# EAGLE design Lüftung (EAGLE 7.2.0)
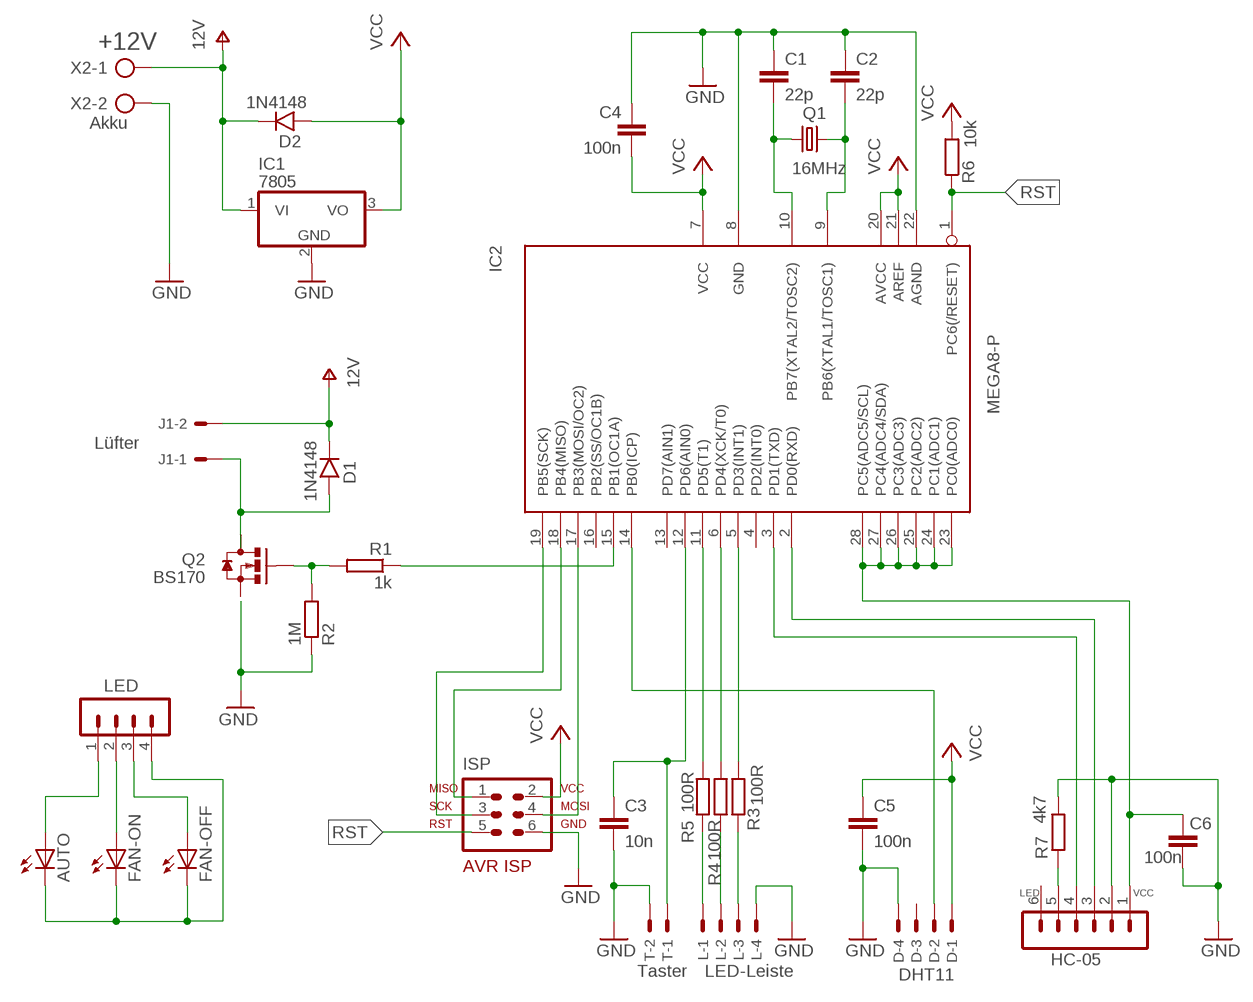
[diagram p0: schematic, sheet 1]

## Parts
AUTO  LED5MM  [LED5MM]
C1  22p  C-EU025-025X050  [C025-025X050]
C2  22p  C-EU025-025X050  [C025-025X050]
C3  10n  C-EU050-030X075  [C050-030X075]
C4  100n  C-EU050-030X075  [C050-030X075]
C5  100n  C-EU050-030X075  [C050-030X075]
C6  100n  C-EU050-030X075  [C050-030X075]
D  DHT11  22-27-2041-04  [6410-04]
D1  1N4148  1N400X.3  [DO41-3]
D2  1N4148  1N400X.3  [DO41-3]
FAN-OFF  LED5MM  [LED5MM]
FAN-ON  LED5MM  [LED5MM]
HC-05  MA06-1  [MA06-1]
IC1  7805  7805TV  [TO220V]
IC2  MEGA8-P  [DIL28-3]
ISP  AVR-ISP-6  [ML6]
J1  Lüfter  22-27-2021-02  [6410-02]
L  LED-Leiste  22-27-2041-04  [6410-04]
LED  MA04-1  [MA04-1]
Q1  16MHz  CRYSTALHC49S  [HC49/S]
Q2  BS170  [SOT54ES]
R1  1k  R-EU_0207/12  [0207/12]
R2  1M  R-EU_0207/2V  [0207/2V]
R3  100R  R-EU_0207/10  [0207/10]
R4  100R  R-EU_0207/10  [0207/10]
R5  100R  R-EU_0207/10  [0207/10]
R6  10k  R-EU_0207/15  [0207/15]
R7  4k7  R-EU_0207/10  [0207/10]
T  Taster  22-27-2021-02  [6410-02]
X2  Akku  AK500/2  [AK500/2]

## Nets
GND: C1.1 C2.1 C3.2 C4.1 C5.2 C6.2 D.4 HC-05.2 IC1.2(GND) IC2.8(GND) IC2.22(AGND) ISP.6 L.4 R2.1 R7.2 T.2 X2.2
N$1: Q2.G R1.2 R2.2
N$2: FAN-ON.A LED.2
N$3: D1.A J1.1
N$4: L.3 R3.1
N$5: L.2 R4.1
N$6: L.1 R5.1
N$7: AUTO.K(C) FAN-OFF.K(C) FAN-ON.K(C) LED.4
N$8: AUTO.A LED.1
N$9: FAN-OFF.A LED.3
N$10: IC2.5(PD3(INT1)) R3.2
N$11: D.2 IC2.14(PB0(ICP))
N$12: C3.1 IC2.12(PD6(AIN0)) T.1
N$14: C1.2 IC2.10(PB7(XTAL2/TOSC2)) Q1.1
N$16: C2.2 IC2.9(PB6(XTAL1/TOSC1)) Q1.2
N$17: HC-05.3 IC2.2(PD0(RXD))
N$18: HC-05.4 IC2.3(PD1(TXD))
N$19: HC-05.5 R7.1
N$20: IC2.6(PD4(XCK/T0)) R4.2
N$21: IC2.18(PB4(MISO)) ISP.1
N$23: IC2.17(PB3(MOSI/OC2)) ISP.4
N$26: C6.1 HC-05.1 IC2.23(PC0(ADC0)) IC2.24(PC1(ADC1)) IC2.25(PC2(ADC2)) IC2.26(PC3(ADC3)) IC2.27(PC4(ADC4/SDA)) IC2.28(PC5(ADC5/SCL))
N$27: IC2.11(PD5(T1)) R5.2
N$28: IC2.15(PB1(OC1A)) R1.1
RST: IC2.1(PC6(/RESET)) ISP.5 R6.1
SCK: IC2.19(PB5(SCK)) ISP.3
V+: D1.C D2.C IC1.1(VI) J1.2 X2.1 ; supply symbol labelled 12V
VCC: C4.2 C5.1 D2.A D.1 IC1.3(VO) IC2.7(VCC) IC2.20(AVCC) IC2.21(AREF) ISP.2 R6.2
Unconnected: D.3 HC-05.6 IC2.4(PD2(INT0)) IC2.13(PD7(AIN1)) IC2.16(PB2(SS/OC1B)) Q2.D Q2.S

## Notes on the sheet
- +12V
- LED | VCC

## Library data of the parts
AUTO FAN-OFF FAN-ON = led:LED: LED
C1-C6 = resistor:C-EU: CAPACITOR, European symbol
D L = con-molex:22-?-04: CONNECTOR wire to board 2.54 mm (.1 inch) pitch header; OC_FARNELL: unknown; OC_NEWARK: unknown
D1 D2 = gm-diodes:1N400X: Rectifier Diodes
HC-05 = con-lstb:MA06-1: PIN HEADER; OC_FARNELL: unknown; OC_NEWARK: unknown
IC1 = linear:78*: Positive VOLTAGE REGULATOR Source: http://cache.national.com/ds/LM/LM78L05.pdf http://www.fairchildsemi.com/ds/LM/LM7805.pdf
IC2 = avr-7:MEGA8-P: MICROCONTROLLER 8 Kbytes FLASH 1 kbytes SRAM 512 bytes EEPROM USART 4-channel 10 bit ADC 2-channel 8 bit ADC
ISP = Ulli:AVR-ISP-6: AVR ISP-6 Serial Programming Header
J1 T = con-molex:22-?-02: CONNECTOR; OC_FARNELL: unknown; OC_NEWARK: unknown
LED = con-lstb:MA04-1: PIN HEADER; OC_FARNELL: unknown; OC_NEWARK: unknown
Q1 = crystal:CRYSTAL: CRYSTAL; OC_FARNELL: 1667008; OC_NEWARK: unknown
Q2 = gm-trans:BS170: N-CHANNEL MOS FET
R1-R7 = resistor:R-EU_: RESISTOR, European symbol
X2 = con-ptr500:AK500/2: CONNECTOR; OC_FARNELL: unknown; OC_NEWARK: unknown

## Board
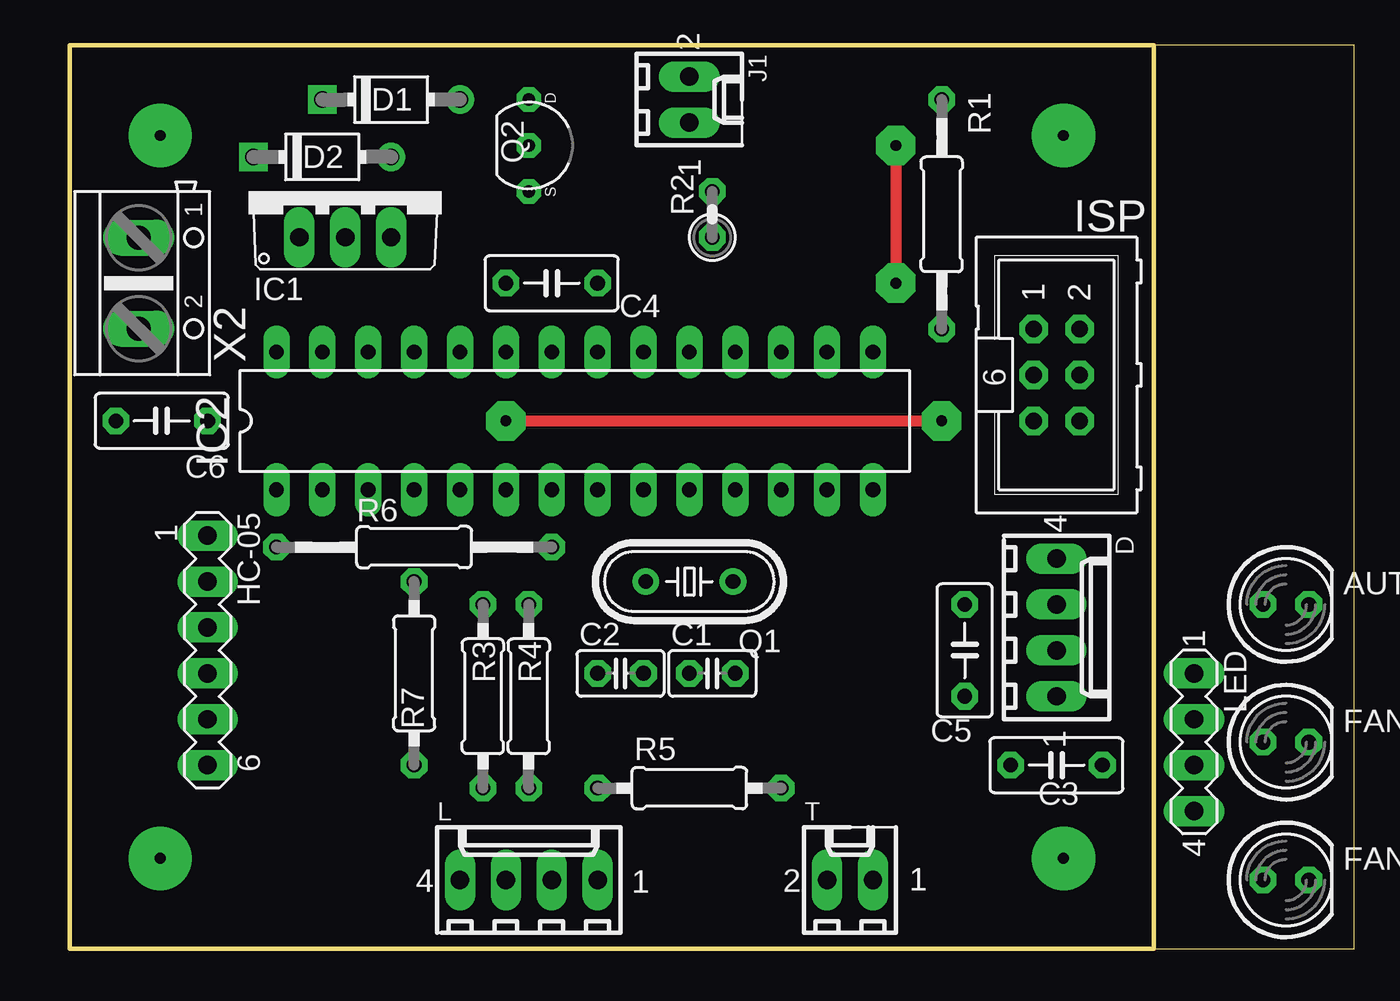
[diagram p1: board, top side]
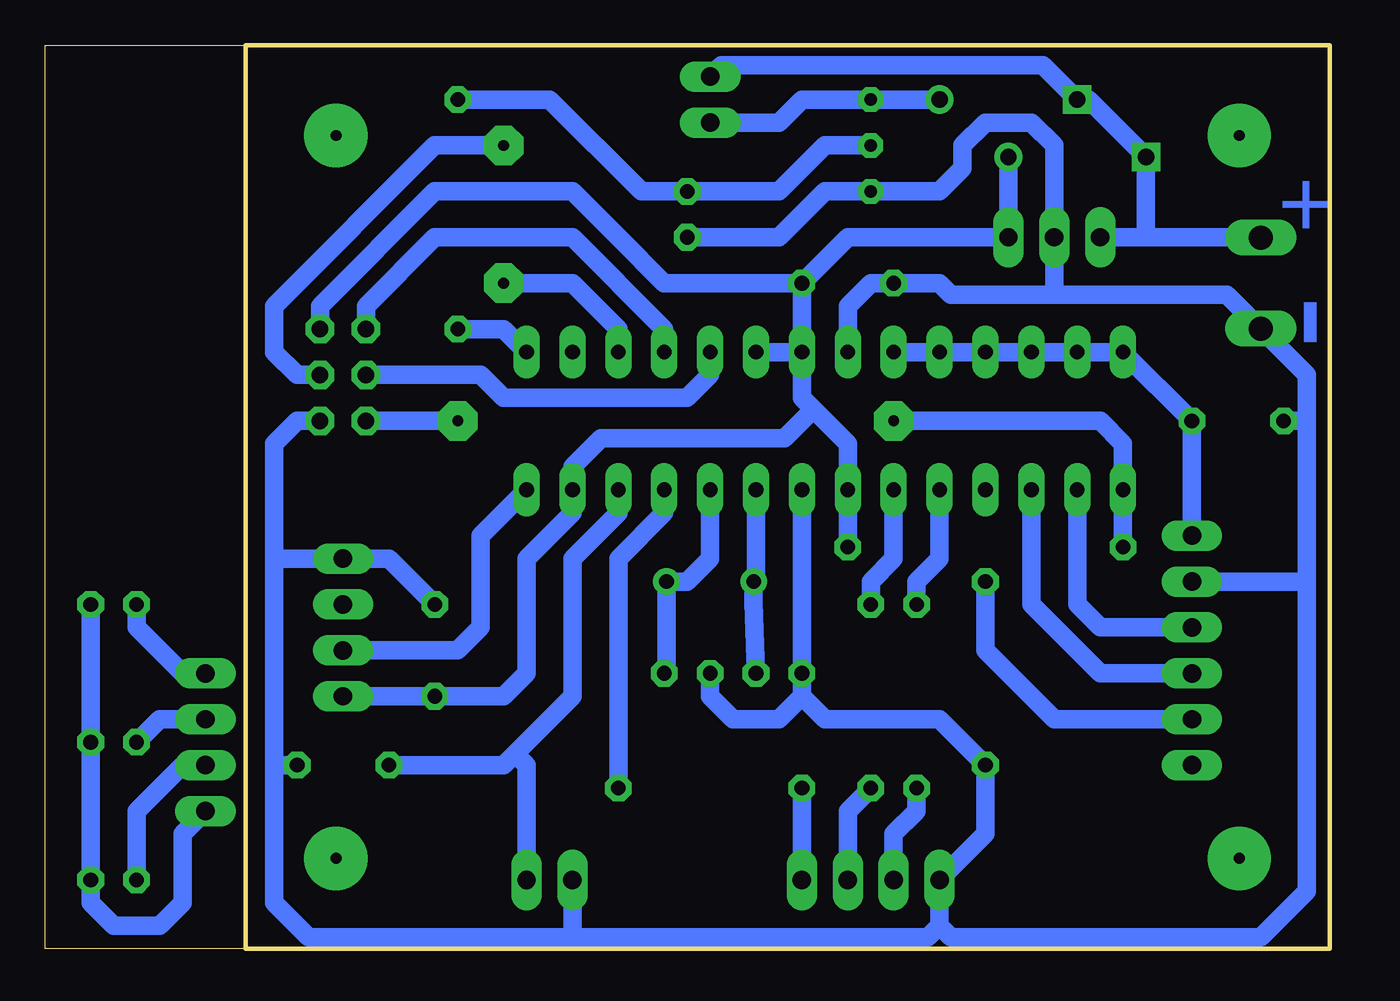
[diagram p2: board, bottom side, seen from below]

Size 71.1 x 50 mm. Coordinates in mm from the lower left corner, seen from the top.
Outline: 60,0 0,0 0,50 60,50
Outline: 60,0 71.1,0 71.1,50 60,50
Outline: 60,50 60,0
Copper layers (1*16): Top 0.035mm / dielectric 1.5mm / Bottom 0.035mm
Design rules "default *": minimum track width 10mil, minimum drill 24mil, track to track 8mil, track to pad 8mil, pad to pad 8mil, via to via 8mil, smd to smd 8mil, copper to edge 40mil, drill to drill 8mil, minimum pad ring 13mil, minimum via ring 8mil, stop-mask expansion 4mil, vias tented up to drill 0mil, thermal gap 10mil

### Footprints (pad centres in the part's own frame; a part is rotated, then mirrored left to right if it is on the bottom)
LED5MM = drill 0.813 octagon: A -1.27,0; K 1.27,0
C025-025X050 = drill 0.813 octagon: 1 -1.27,0; 2 1.27,0
C050-030X075 = drill 0.813 octagon: 1 -2.54,0; 2 2.54,0
6410-04 = drill 1.016 long: 1 3.81,0; 2 1.27,0; 3 -1.27,0; 4 -3.81,0
DO41-3 = drill 0.9: A 3.81,0 | drill 0.9 square: C -3.81,0
MA06-1 = drill 1.016 long: 1 -6.35,0; 2 -3.81,0; 3 -1.27,0; 4 1.27,0; 5 3.81,0; 6 6.35,0
TO220V = drill 1.016 long: 1 -2.54,-2.54; 2 0,-2.54; 3 2.54,-2.54
DIL28-3 = drill 0.813 long: 1 -16.51,-3.81; 2 -13.97,-3.81; 3 -11.43,-3.81; 4 -8.89,-3.81; 5 -6.35,-3.81; 6 -3.81,-3.81; 7 -1.27,-3.81; 8 1.27,-3.81; 9 3.81,-3.81; 10 6.35,-3.81; 11 8.89,-3.81; 12 11.43,-3.81; 13 13.97,-3.81; 14 16.51,-3.81; 15 16.51,3.81; 16 13.97,3.81; 17 11.43,3.81; 18 8.89,3.81; 19 6.35,3.81; 20 3.81,3.81; 21 1.27,3.81; 22 -1.27,3.81; 23 -3.81,3.81; 24 -6.35,3.81; 25 -8.89,3.81; 26 -11.43,3.81; 27 -13.97,3.81; 28 -16.51,3.81
ML6 = drill 0.914 octagon: 1 -2.54,-1.27; 2 -2.54,1.27; 3 0,-1.27; 4 0,1.27; 5 2.54,-1.27; 6 2.54,1.27
6410-02 = drill 1.016 long: 1 1.27,0; 2 -1.27,0
MA04-1 = drill 1.016 long: 1 -3.81,0; 2 -1.27,0; 3 1.27,0; 4 3.81,0
HC49/S = drill 0.813: 1 -2.413,0; 2 2.413,0
SOT54ES = drill 0.7 octagon: D -2.54,0; G 0,0; S 2.54,0
0207/12 = drill 0.813 octagon: 1 -6.35,0; 2 6.35,0
0207/2V = drill 0.813 octagon: 1 -1.27,0; 2 1.27,0
0207/10 = drill 0.813 octagon: 1 -5.08,0; 2 5.08,0
0207/15 = drill 0.813 octagon: 1 -7.62,0; 2 7.62,0
AK500/2 = drill 1.321 long: 1 -2.515,0; 2 2.515,0

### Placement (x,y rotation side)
AUTO  67.31,19.05 0 top
C1  35.56,15.24 0 top
C2  30.48,15.24 0 top
C3  54.61,10.16 0 top
C4  26.67,36.83 0 top
C5  49.53,16.51 90 top
C6  5.08,29.21 180 top
D  54.61,17.78 270 top
D1  17.78,46.99 0 top
D2  13.97,43.81 0 top
FAN-OFF  67.31,3.81 0 top
FAN-ON  67.31,11.43 0 top
HC-05  7.62,16.51 270 top
IC1  15.24,41.91 0 top
IC2  27.94,29.21 0 top
ISP  54.61,31.75 270 top
J1  34.29,46.99 270 top
L  25.4,3.81 0 top
LED  62.23,11.43 270 top
Q1  34.29,20.32 180 top
Q2  25.4,44.45 270 top
R1  48.26,40.64 90 top
R2  35.56,40.64 90 top
R3  22.86,13.97 90 top
R4  25.4,13.97 90 top
R5  34.29,8.89 0 top
R6  19.05,22.23 0 top
R7  19.05,15.24 270 top
T  43.18,3.81 0 top
X2  3.81,36.83 270 top

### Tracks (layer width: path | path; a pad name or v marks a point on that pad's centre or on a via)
GND
  Bottom 1.016: 41.91,0.64 22.23,0.64 21.59,1.27 | 41.91,0.64 56.52,0.64 58.42,2.54 58.42,10.16 | C5.2 52.07,21.59 D.4 58.42,21.59 | C1.1 34.29,13.97 33.02,12.7 30.48,12.7 29.21,13.97 | 29.21,13.97 C2.1 IC2.8 | X2.2 1.27,31.77 1.27,29.21 | ISP.6 57.15,29.21 58.42,27.94 58.42,21.59 | 58.42,10.16 58.42,21.59 | HC-05.2 1.27,20.32 | C3.2 58.42,10.16 | 1.27,20.32 1.27,3.17 3.81,0.64 20.95,0.64 21.59,1.27 | 29.21,13.97 27.94,12.7 21.59,12.7 R7.2 19.05,6.35 L.4 21.59,1.27 | 5.08,34.29 3.83,34.29 X2.2 | 1.27,20.32 1.27,29.21 | C6.2 1.27,29.21 | T.2 41.91,0.64 | 15.24,36.2 20.95,36.2 21.59,36.83 C4.1 25.4,36.83 26.67,35.56 IC2.22 | 15.24,36.2 5.69,36.2 X2.2 | 15.24,36.2 IC1.2 15.24,44.45 16.51,45.72 19.05,45.72 20.32,44.45 20.32,43.18 21.59,41.91 27.94,41.91 30.48,39.37 R2.1
N$1
  Bottom 1.016: R1.2 43.18,46.99 38.1,41.91 R2.2 30.48,41.91 27.94,44.45 Q2.G
N$2
  Bottom 1.016: FAN-ON.A 64.77,12.7 LED.2
N$3
  Bottom 1.016: J1.1 30.48,45.72 29.21,46.99 D1.A
N$4
  Bottom 1.016: L.3 24.13,6.35 22.86,7.62 R3.1
N$5
  Bottom 1.016: L.2 26.67,7.62 R4.1
N$6
  Bottom 1.016: L.1 R5.1
N$7
  Bottom 1.016: LED.4 63.5,6.35 63.5,2.54 64.77,1.27 67.31,1.27 68.58,2.54 FAN-OFF.K FAN-ON.K AUTO.K
N$8
  Bottom 1.016: AUTO.A 66.04,17.78 63.5,15.24 LED.1
N$9
  Bottom 1.016: LED.3 63.5,10.16 66.04,7.62 FAN-OFF.A
N$10
  Bottom 1.016: R3.2 22.86,20.32 21.59,21.59 IC2.5
N$11
  Bottom 1.016: D.2 48.26,16.51 46.99,17.78 46.99,22.86 IC2.14
N$12
  Bottom 1.016: C3.1 45.72,10.16 45.09,10.79 | 45.09,10.79 41.91,13.97 41.91,21.59 39.37,24.13 IC2.12 | T.1 44.45,10.16 45.09,10.79
N$13  (via drill 0.6 pad 3.5)
  other vias: 5,5
N$14
  Bottom 1.016: C1.2 36.7,15.37 Q1.1 35.56,20.32 34.29,21.59 IC2.10
N$15  (via drill 0.6 pad 3.5)
  other vias: 55,45
N$16
  Bottom 1.016: IC2.9 31.75,20.45 Q1.2 31.88,19.18 C2.2
N$17
  Bottom 1.016: IC2.2 13.97,19.05 12.7,17.78 HC-05.3
N$18
  Bottom 1.016: IC2.3 16.51,19.05 12.7,15.24 HC-05.4
N$19
  Bottom 1.016: HC-05.5 15.24,12.7 19.05,16.51 R7.1
N$20
  Bottom 1.016: R4.2 25.4,20.32 24.13,21.59 IC2.6
N$21
  Bottom 1.016: ISP.1 53.34,35.56 49.53,39.37 41.91,39.37 36.83,34.29 IC2.18
N$23  (via drill 0.6 pad 2.18)
  Top 0.61: v45.72,44.45 v45.72,36.83
  Bottom 1.016: ISP.4 57.15,31.75 58.42,33.02 58.42,35.56 49.53,44.45 v45.72,44.45 | IC2.17 39.37,34.29 41.91,36.83 v45.72,36.83
N$24  (via drill 0.6 pad 3.5)
  other vias: 55,5
N$25  (via drill 0.6 pad 3.5)
  other vias: 5,45
N$26
  Bottom 1.016: HC-05.1 C6.1 IC2.28 IC2.27 IC2.26 IC2.25 IC2.24 IC2.23
N$27
  Bottom 1.016: R5.2 39.37,21.59 36.83,24.13 IC2.11
N$28
  Bottom 1.016: IC2.15 45.72,34.29 R1.1
RST  (via drill 0.6 pad 2.18)
  Top 0.61: v24.13,29.21 v48.26,29.21
  Bottom 1.016: R6.1 IC2.1 11.43,27.94 12.7,29.21 v24.13,29.21 | v48.26,29.21 ISP.5
SCK
  Bottom 1.016: ISP.3 46.99,31.75 45.72,30.48 35.56,30.48 34.29,31.75 IC2.19
V+
  Bottom 1.016: IC1.1 10.16,39.37 | 10.16,39.37 3.83,39.37 X2.1 | 10.16,39.37 D2.C 13.34,46.99 D1.C 15.88,48.9 33.66,48.9 J1.2
VCC
  Bottom 0.61: IC2.7 26.67,26.67
  Bottom 1.016: IC2.21 IC2.20 | C4.2 26.67,39.37 IC1.3 D2.A | D.1 C5.1 45.72,13.97 44.45,15.24 44.45,21.59 41.91,24.13 41.91,25.4 41.91,26.67 40.32,28.26 30.16,28.26 28.57,29.84 | R6.2 IC2.7 26.67,27.94 28.57,29.84 | ISP.2 55.88,35.56 49.53,41.91 41.91,41.91 39.37,39.37 36.83,36.83 C4.2 | IC2.21 29.21,30.48 28.57,29.84 | C4.2 IC2.21

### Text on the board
Bottom: + | -
tTest: Lüfter | Akku | HC-05 | DHT11 | Taster | LED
